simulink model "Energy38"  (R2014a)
settings: Solver=VariableStepDiscrete  StartTime=0.0  StopTime=0.1  RelTol=1e-3
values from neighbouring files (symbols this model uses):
  Gsimulated = Ivertical4'    [main.m]
libraries: fl_lib x56, nesl_utility x29, elec_lib x25

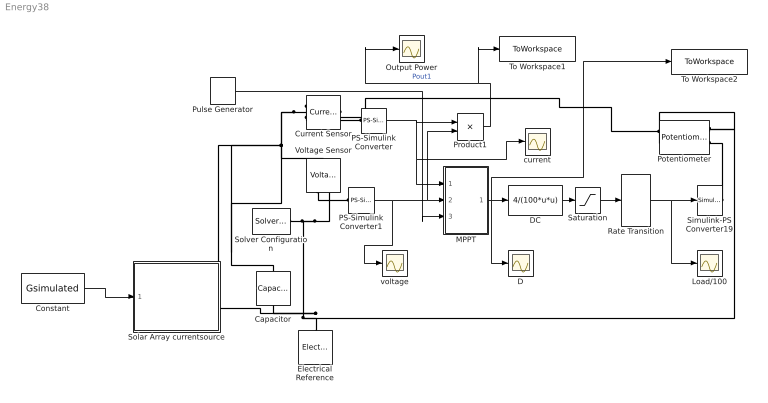
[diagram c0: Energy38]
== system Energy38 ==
  Capacitor : fl_lib/Electrical/Electrical Elements/Capacitor  c=1e-6 F  r=1e-6 Ohm  g=0 1/Ohm  i_specify=off  i_priority=High  i=0 A  v_specify=off  v_priority=High  v=0 V  vc_specify=off  vc_priority=High  vc=0 V
  Constant : Constant  Value=Gsimulated
  Current Sensor : fl_lib/Electrical/Electrical Sensors/Current Sensor
  D : Scope
  DC : Fcn  Expr=4/(100*u*u)
  Electrical Reference : fl_lib/Electrical/Electrical Elements/Electrical Reference
  Load/100 : Scope
  MPPT : Subsystem
  Output Power : Scope
  PS-Simulink Converter : nesl_utility/PS-Simulink Converter  PhysicalDomain=network_engine_domain  SubClassName=ps_output  LeftPortType=input  RightPortType=output  PseudoPeriodic=off  Frequencies=[]  Unit=1  AffineConversion=off
  PS-Simulink Converter1 : nesl_utility/PS-Simulink Converter  PhysicalDomain=network_engine_domain  SubClassName=ps_output  LeftPortType=input  RightPortType=output  PseudoPeriodic=off  Frequencies=[]  Unit=1  AffineConversion=off
  Potentiometer : elec_lib/Passive Devices/Potentiometer  R0=100 Ohm  Rw=0.01 Ohm  Rcenter=200 Ohm  xmin=0  xmax=1  Taper=1  Gradient=1  xminL=0  xmaxL=1  lambda=1  A=1 Ohm
  Product1 : Product
  Pulse Generator : DiscretePulseGenerator  PulseType=Time based  Period=0.3  PulseWidth=0.1
  Rate Transition : RateTransition
  Saturation : Saturate  UpperLimit=1  LowerLimit=0
  Simulink-PS Converter19 : nesl_utility/Simulink-PS Converter  PhysicalDomain=network_engine_domain  SubClassName=ps_input  LeftPortType=input  RightPortType=output  PseudoPeriodic=off  Frequencies=[]  NoiseDistribution=none  NoiseParameters=[]  Unit=1  AffineConversion=off  InputFiltering=off  SimscapeFilterOrder=1  InputFilterTimeConstant=0.001  UdotUserProvided=1
  Solar Array currentsource : Subsystem
  Solver Configuration : nesl_utility/Solver Configuration  PhysicalDomain=network_engine_domain  SubClassName=solver  LeftPortType=input  RightPortType=generic  Accelerate=off  Tones=[]  Harmonics=[]  SimulateNoise=off  Profile=off  UseLocalSampling=off  EnableSwitchedLinearOptims=on  FrequencyDomain=off  UseCCode=off  RelTol=0.001  AbsTol=1e-06  MinStep=1e-09  ToWorkspace=off  DoDC=off  ResidualTolerance=1e-09  UseLocalSolver=on  LocalSolverChoice=NE_BACKWARD_EULER_ADVANCER  LocalSolverSampleTime=1e-4  DoFixedCost=on  MaxNonlinIter=3  MaxModeIter=2  LinearAlgebra=Sparse  DelaysMemoryBudget=1024  AutomaticFiltering=on  FilteringTimeConstant=0.001
  To Workspace1 : ToWorkspace  VariableName=Psimulated  SampleTime=-1
  To Workspace2 : ToWorkspace  VariableName=Dsimulated  SampleTime=-1
  Voltage Sensor : fl_lib/Electrical/Electrical Sensors/Voltage Sensor
  current : Scope
  voltage : Scope
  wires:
  Product1/1 -> Output Power/1, To Workspace1/1  "Pout1"
  DC/1 -> Saturation/1
  Saturation/1 -> Rate Transition/1
  MPPT/1(D) -> To Workspace2/1, D/1, DC/1
  Rate Transition/1 -> Load/100/1, Simulink-PS Converter19/1
  PS-Simulink Converter1/1 -> voltage/1, Product1/2, MPPT/2(V)
  Pulse Generator/1 -> MPPT/3(Control)
  PS-Simulink Converter/1 -> current/1, MPPT/1(I), Product1/1
  Constant/1 -> Solar Array currentsource/1(Gsimulated)
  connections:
  Current Sensor/LConn1 -- Voltage Sensor/LConn1 -- Capacitor/LConn1 -- Solar Array currentsource/RConn1
  Solver Configuration/RConn1 -- Voltage Sensor/RConn2 -- Capacitor/RConn1 -- Solar Array currentsource/RConn2 -- Potentiometer/LConn2 -- Potentiometer/RConn1 -- Electrical Reference/LConn1
  Voltage Sensor/RConn1 -- PS-Simulink Converter1/LConn1
  Current Sensor/RConn1 -- PS-Simulink Converter/LConn1
  Simulink-PS Converter19/RConn1 -- Potentiometer/RConn2
  Potentiometer/LConn1 -- Current Sensor/RConn2

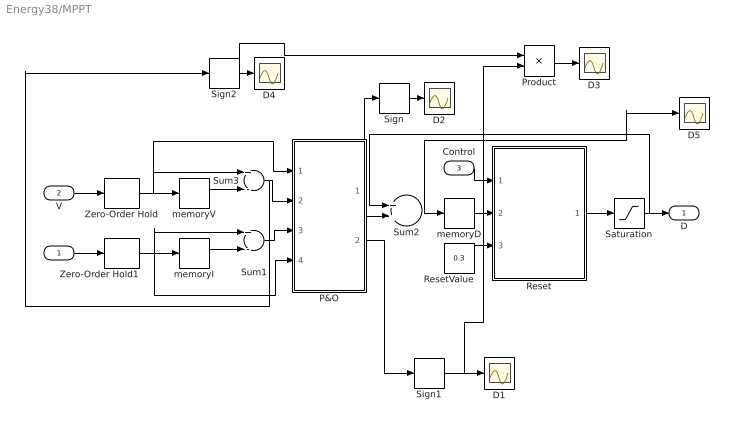
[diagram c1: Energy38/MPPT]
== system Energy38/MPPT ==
  I : Inport
  V : Inport  Port=2
  Control : Inport  Port=3
  D{1..5} (5 alike) : Scope
  P&O : MATLAB Function  TreatAsAtomicUnit=on
  Product : Product
  Reset : MATLAB Function  TreatAsAtomicUnit=on
  ResetValue : Constant  Value=0.3
  Saturation : Saturate  UpperLimit=1  LowerLimit=0
  Sign : Signum
  Sign1 : Signum
  Sign2 : Signum
  Sum1 : Sum  Inputs=+-
  Sum2 : Sum  Inputs=2
  Sum3 : Sum  Inputs=+-
  Zero-Order Hold : ZeroOrderHold  SampleTime=1e-3
  Zero-Order Hold1 : ZeroOrderHold  SampleTime=1e-3
  memoryD : Memory  X0=0.3  InheritSampleTime=on
  memoryI : Memory  InheritSampleTime=on
  memoryV : Memory  InheritSampleTime=on
  D : Outport
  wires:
  Sum2/1 -> D5/1, memoryD/1
  V/1 -> Zero-Order Hold/1
  I/1 -> Zero-Order Hold1/1
  Zero-Order Hold/1 -> P&O/1(V), Sum3/1, memoryV/1
  memoryV/1 -> Sum3/2
  Zero-Order Hold1/1 -> Sum1/1, P&O/4(I), memoryI/1
  memoryI/1 -> Sum1/2
  Saturation/1 -> Sum2/1, D/1
  Sum3/1 -> Sign2/1, P&O/2(dV)
  Sum1/1 -> P&O/3(dI)
  P&O/1(dD) -> Sum2/2, Sign/1
  ResetValue/1 -> Reset/3(ResetValue)
  memoryD/1 -> Reset/2(in)
  Reset/1(out) -> Saturation/1
  Control/1 -> Reset/1(control)
  Sign/1 -> D2/1
  Sign1/1 -> Product/2, D1/1
  P&O/2(dP) -> Sign1/1
  Product/1 -> D3/1
  Sign2/1 -> Product/1, D4/1

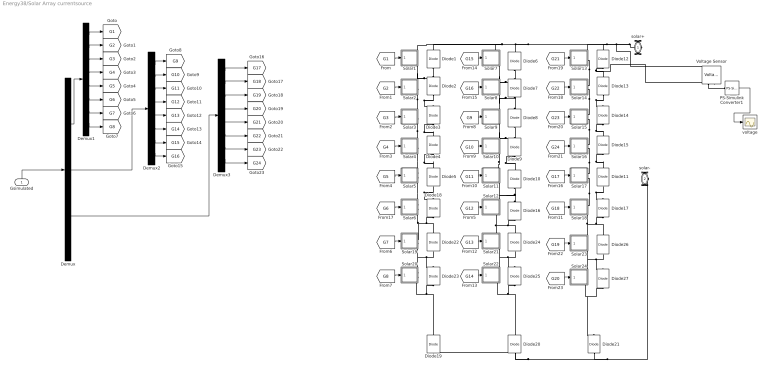
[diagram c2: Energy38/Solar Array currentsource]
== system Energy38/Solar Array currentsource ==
  Gsimulated : Inport
  Demux : Demux  Outputs=3
  Demux1 : Demux  Outputs=8
  Demux2 : Demux  Outputs=8
  Demux3 : Demux  Outputs=8
  Diode{1..27} (27 alike) : fl_lib/Electrical/Electrical Elements/Diode  Vf=0.1 mV  Ron=0.6 Ohm  Goff=1e-10 1/Ohm  i_specify=off  i_priority=High  i=0 A  v_specify=off  v_priority=High  v=0 V
  PS-Simulink Converter1 : nesl_utility/PS-Simulink Converter  PhysicalDomain=network_engine_domain  SubClassName=ps_output  LeftPortType=input  RightPortType=output  PseudoPeriodic=off  Frequencies=[]  Unit=1  AffineConversion=off
  Solar1 : Subsystem
  Solar10 : Subsystem
  Solar11 : Subsystem
  Solar12 : Subsystem
  Solar13 : Subsystem
  Solar14 : Subsystem
  Solar15 : Subsystem
  Solar16 : Subsystem
  Solar17 : Subsystem
  Solar18 : Subsystem
  Solar19 : Subsystem
  Solar2 : Subsystem
  Solar20 : Subsystem
  Solar21 : Subsystem
  Solar22 : Subsystem
  Solar23 : Subsystem
  Solar24 : Subsystem
  Solar3 : Subsystem
  Solar4 : Subsystem
  Solar5 : Subsystem
  Solar6 : Subsystem
  Solar7 : Subsystem
  Solar8 : Subsystem
  Solar9 : Subsystem
  Voltage Sensor : fl_lib/Electrical/Electrical Sensors/Voltage Sensor
  voltage : Scope
  solar+ : PMIOPort  Port=1  Side=Right
  solar- : PMIOPort  Port=2  Side=Right
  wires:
  [G1] -> Solar1/1(G)
  [G2] -> Solar2/1(G)
  [G3] -> Solar3/1(G)
  Gsimulated/1 -> Demux/1
  [G4] -> Solar4/1(G)
  [G9] -> Solar9/1(G)
  [G10] -> Solar10/1(G)
  [G11] -> Solar11/1(G)
  [G17] -> Solar17/1(G)
  Demux/1 -> Demux1/1
  Demux1/1 -> [G1]
  Demux1/2 -> [G2]
  Demux1/3 -> [G3]
  Demux1/4 -> [G4]
  Demux1/5 -> [G5]
  Demux1/6 -> [G6]
  Demux/2 -> Demux2/1
  Demux/3 -> Demux3/1
  [G6] -> Solar6/1(G)
  [G12] -> Solar12/1(G)
  [G18] -> Solar18/1(G)
  [G5] -> Solar5/1(G)
  PS-Simulink Converter1/1 -> voltage/1
  Demux1/7 -> [G7]
  Demux1/8 -> [G8]
  Demux2/1 -> [G9]
  Demux2/2 -> [G10]
  Demux2/3 -> [G11]
  Demux2/4 -> [G12]
  Demux2/5 -> [G13]
  Demux2/6 -> [G14]
  Demux2/7 -> [G15]
  Demux2/8 -> [G16]
  Demux3/1 -> [G17]
  Demux3/2 -> [G18]
  Demux3/3 -> [G19]
  Demux3/4 -> [G20]
  Demux3/5 -> [G21]
  Demux3/6 -> [G22]
  Demux3/7 -> [G23]
  Demux3/8 -> [G24]
  [G7] -> Solar19/1(G)
  [G8] -> Solar20/1(G)
  [G19] -> Solar23/1(G)
  [G20] -> Solar24/1(G)
  [G13] -> Solar21/1(G)
  [G14] -> Solar22/1(G)
  [G15] -> Solar7/1(G)
  [G16] -> Solar8/1(G)
  [G21] -> Solar13/1(G)
  [G22] -> Solar14/1(G)
  [G23] -> Solar15/1(G)
  [G24] -> Solar16/1(G)
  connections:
  Solar15/RConn2 -- Diode15/RConn1 -- Diode14/LConn1 -- Solar16/RConn1
  Solar13/RConn2 -- Voltage Sensor/RConn2 -- Diode13/RConn1 -- Diode12/LConn1 -- Solar14/RConn1
  Diode7/LConn1 -- Diode8/RConn1 -- Solar9/RConn1 -- Solar8/RConn2
  Solar4/RConn2 -- Diode5/RConn1 -- Diode4/LConn1 -- Solar5/RConn1
  solar+/RConn1 -- Solar1/RConn1 -- Diode1/RConn1 -- Solar7/RConn1 -- Diode6/RConn1 -- Solar13/RConn1 -- Diode12/RConn1 -- Voltage Sensor/LConn1
  Diode2/RConn1 -- Diode1/LConn1 -- Solar1/RConn2 -- Solar2/RConn1
  Diode7/RConn1 -- Diode6/LConn1 -- Solar7/RConn2 -- Solar8/RConn1
  Solar14/RConn2 -- Diode13/LConn1 -- Diode14/RConn1 -- Solar15/RConn1
  Solar2/RConn2 -- Diode2/LConn1 -- Diode3/RConn1 -- Solar3/RConn1
  Solar3/RConn2 -- Diode4/RConn1 -- Diode3/LConn1 -- Solar4/RConn1
  Diode9/RConn1 -- Diode8/LConn1 -- Solar9/RConn2 -- Solar10/RConn1
  Solar17/RConn1 -- Diode11/RConn1 -- Diode15/LConn1 -- Solar16/RConn2
  Solar10/RConn2 -- Solar11/RConn1 -- Diode10/RConn1 -- Diode9/LConn1
  Diode16/RConn1 -- Diode10/LConn1 -- Solar11/RConn2 -- Solar12/RConn1
  Solar6/RConn1 -- Diode5/LConn1 -- Diode18/RConn1 -- Solar5/RConn2
  Solar12/RConn2 -- Solar21/RConn1 -- Diode24/RConn1 -- Diode16/LConn1
  Solar18/RConn1 -- Diode11/LConn1 -- Diode17/RConn1 -- Solar17/RConn2
  solar-/RConn1 -- Diode21/LConn1 -- Diode20/LConn1 -- Diode19/LConn1
  Solar18/RConn2 -- Solar23/RConn1 -- Diode17/LConn1 -- Diode26/RConn1
  Voltage Sensor/RConn1 -- PS-Simulink Converter1/LConn1
  Solar6/RConn2 -- Solar19/RConn1 -- Diode22/RConn1 -- Diode18/LConn1
  Solar20/RConn2 -- Diode19/RConn1 -- Diode23/LConn1
  Solar19/RConn2 -- Diode22/LConn1 -- Diode23/RConn1 -- Solar20/RConn1
  Solar22/RConn2 -- Diode20/RConn1 -- Diode25/LConn1
  Solar21/RConn2 -- Diode24/LConn1 -- Diode25/RConn1 -- Solar22/RConn1
  Solar24/RConn2 -- Diode27/LConn1 -- Diode21/RConn1
  Solar23/RConn2 -- Diode26/LConn1 -- Diode27/RConn1 -- Solar24/RConn1

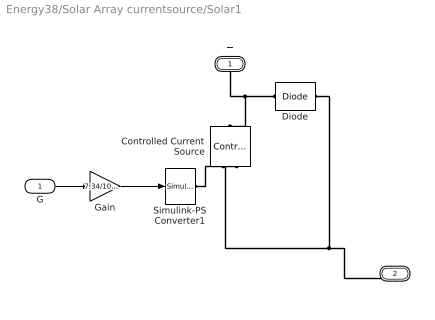
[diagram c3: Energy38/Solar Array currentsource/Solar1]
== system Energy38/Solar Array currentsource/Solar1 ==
  G : Inport
  Controlled Current Source : fl_lib/Electrical/Electrical Sources/Controlled Current Source
  Diode : elec_lib/Semiconductor Devices/Diode  ModelType=3  Vf=0.6 V  Ron=0.3 Ohm  Goff=1e-8 S  Rz=0.3 Ohm  Vz=50 V  C_PWL=5 pF  prmExp=2  I12=[ 0.0137 0.545 ] A  V12=[ 0.6 0.7 ] V  I1=0.0137 A  V1=0.6 V  RS=0.01 Ohm  IS=1.2614e-07 A  Tmeas=25 C  ec=117.5087  BV=Inf V  C_param=1  CJ0=5 pF  VJ=1 V  Mgrad=0.5  Vvec=[ 0.1 10 100 ] V  Cvec=[ 3.5 1 0.4 ] pF  FC=0.5  Q_param=1  Irrm=-7.15 A  iF=4 A  didt=-750 A/us  trr=115 ns  TT=50 ns  tau=100 ns  T_param=1  IS_T2=1.25e-7 A  I1_T2=0.245 A  V1_T2=0.5 V  Tmeas2=125 C  EG_param=1  EG=1.11 eV  XTI_param=1  XTI=3  dBVdT=0 V/K  Tdevice=25 C  Rth=[ 0 10 ] K/W  thermal_mass_parameterization=1  thermal_mass=[ 0 1 ] J/K  thermal_time_constant=[ 0 10 ] s  thermal_mass_initial_temperatures=[ 25 25 ] C
  Gain : Gain  Gain=7.34/1000
  Simulink-PS Converter1 : nesl_utility/Simulink-PS Converter  PhysicalDomain=network_engine_domain  SubClassName=ps_input  LeftPortType=input  RightPortType=output  PseudoPeriodic=off  Frequencies=[]  NoiseDistribution=none  NoiseParameters=[]  Unit=1  AffineConversion=off  InputFiltering=off  SimscapeFilterOrder=1  InputFilterTimeConstant=0.001  UdotUserProvided=1
  + : PMIOPort  Port=1  Side=Right
  - : PMIOPort  Port=2  Side=Right
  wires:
  G/1 -> Gain/1
  Gain/1 -> Simulink-PS Converter1/1
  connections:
  Simulink-PS Converter1/RConn1 -- Controlled Current Source/RConn1
  Diode/RConn1 -- -/RConn1 -- Controlled Current Source/RConn2
  Diode/LConn1 -- Controlled Current Source/LConn1 -- +/RConn1

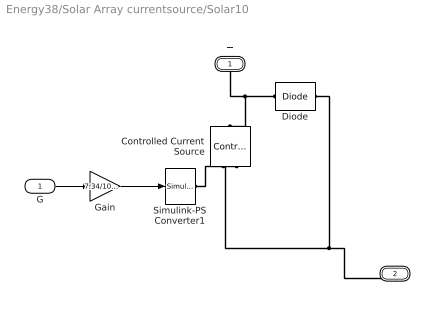
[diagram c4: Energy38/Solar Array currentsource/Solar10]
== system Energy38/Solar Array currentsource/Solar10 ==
  G : Inport
  Controlled Current Source : fl_lib/Electrical/Electrical Sources/Controlled Current Source
  Diode : elec_lib/Semiconductor Devices/Diode  ModelType=3  Vf=0.6 V  Ron=0.3 Ohm  Goff=1e-8 S  Rz=0.3 Ohm  Vz=50 V  C_PWL=5 pF  prmExp=2  I12=[ 0.0137 0.545 ] A  V12=[ 0.6 0.7 ] V  I1=0.0137 A  V1=0.6 V  RS=0.01 Ohm  IS=1.2614e-07 A  Tmeas=25 C  ec=117.5087  BV=Inf V  C_param=1  CJ0=5 pF  VJ=1 V  Mgrad=0.5  Vvec=[ 0.1 10 100 ] V  Cvec=[ 3.5 1 0.4 ] pF  FC=0.5  Q_param=1  Irrm=-7.15 A  iF=4 A  didt=-750 A/us  trr=115 ns  TT=50 ns  tau=100 ns  T_param=1  IS_T2=1.25e-7 A  I1_T2=0.245 A  V1_T2=0.5 V  Tmeas2=125 C  EG_param=1  EG=1.11 eV  XTI_param=1  XTI=3  dBVdT=0 V/K  Tdevice=25 C  Rth=[ 0 10 ] K/W  thermal_mass_parameterization=1  thermal_mass=[ 0 1 ] J/K  thermal_time_constant=[ 0 10 ] s  thermal_mass_initial_temperatures=[ 25 25 ] C
  Gain : Gain  Gain=7.34/1000
  Simulink-PS Converter1 : nesl_utility/Simulink-PS Converter  PhysicalDomain=network_engine_domain  SubClassName=ps_input  LeftPortType=input  RightPortType=output  PseudoPeriodic=off  Frequencies=[]  NoiseDistribution=none  NoiseParameters=[]  Unit=1  AffineConversion=off  InputFiltering=off  SimscapeFilterOrder=1  InputFilterTimeConstant=0.001  UdotUserProvided=1
  + : PMIOPort  Port=1  Side=Right
  - : PMIOPort  Port=2  Side=Right
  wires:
  G/1 -> Gain/1
  Gain/1 -> Simulink-PS Converter1/1
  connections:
  Simulink-PS Converter1/RConn1 -- Controlled Current Source/RConn1
  Diode/RConn1 -- -/RConn1 -- Controlled Current Source/RConn2
  Diode/LConn1 -- Controlled Current Source/LConn1 -- +/RConn1

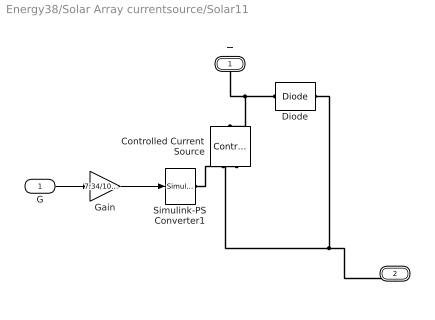
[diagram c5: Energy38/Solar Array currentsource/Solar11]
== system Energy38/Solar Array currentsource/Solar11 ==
  G : Inport
  Controlled Current Source : fl_lib/Electrical/Electrical Sources/Controlled Current Source
  Diode : elec_lib/Semiconductor Devices/Diode  ModelType=3  Vf=0.6 V  Ron=0.3 Ohm  Goff=1e-8 S  Rz=0.3 Ohm  Vz=50 V  C_PWL=5 pF  prmExp=2  I12=[ 0.0137 0.545 ] A  V12=[ 0.6 0.7 ] V  I1=0.0137 A  V1=0.6 V  RS=0.01 Ohm  IS=1.2614e-07 A  Tmeas=25 C  ec=117.5087  BV=Inf V  C_param=1  CJ0=5 pF  VJ=1 V  Mgrad=0.5  Vvec=[ 0.1 10 100 ] V  Cvec=[ 3.5 1 0.4 ] pF  FC=0.5  Q_param=1  Irrm=-7.15 A  iF=4 A  didt=-750 A/us  trr=115 ns  TT=50 ns  tau=100 ns  T_param=1  IS_T2=1.25e-7 A  I1_T2=0.245 A  V1_T2=0.5 V  Tmeas2=125 C  EG_param=1  EG=1.11 eV  XTI_param=1  XTI=3  dBVdT=0 V/K  Tdevice=25 C  Rth=[ 0 10 ] K/W  thermal_mass_parameterization=1  thermal_mass=[ 0 1 ] J/K  thermal_time_constant=[ 0 10 ] s  thermal_mass_initial_temperatures=[ 25 25 ] C
  Gain : Gain  Gain=7.34/1000
  Simulink-PS Converter1 : nesl_utility/Simulink-PS Converter  PhysicalDomain=network_engine_domain  SubClassName=ps_input  LeftPortType=input  RightPortType=output  PseudoPeriodic=off  Frequencies=[]  NoiseDistribution=none  NoiseParameters=[]  Unit=1  AffineConversion=off  InputFiltering=off  SimscapeFilterOrder=1  InputFilterTimeConstant=0.001  UdotUserProvided=1
  + : PMIOPort  Port=1  Side=Right
  - : PMIOPort  Port=2  Side=Right
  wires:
  G/1 -> Gain/1
  Gain/1 -> Simulink-PS Converter1/1
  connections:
  Simulink-PS Converter1/RConn1 -- Controlled Current Source/RConn1
  Diode/RConn1 -- -/RConn1 -- Controlled Current Source/RConn2
  Diode/LConn1 -- Controlled Current Source/LConn1 -- +/RConn1

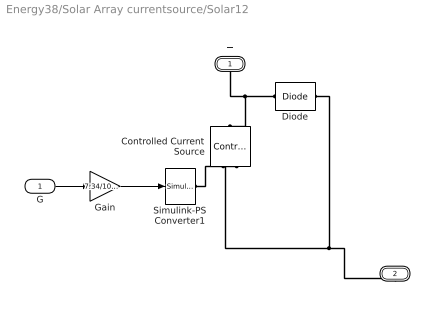
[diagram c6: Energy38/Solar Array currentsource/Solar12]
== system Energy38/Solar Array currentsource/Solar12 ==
  G : Inport
  Controlled Current Source : fl_lib/Electrical/Electrical Sources/Controlled Current Source
  Diode : elec_lib/Semiconductor Devices/Diode  ModelType=3  Vf=0.6 V  Ron=0.3 Ohm  Goff=1e-8 S  Rz=0.3 Ohm  Vz=50 V  C_PWL=5 pF  prmExp=2  I12=[ 0.0137 0.545 ] A  V12=[ 0.6 0.7 ] V  I1=0.0137 A  V1=0.6 V  RS=0.01 Ohm  IS=1.2614e-07 A  Tmeas=25 C  ec=117.5087  BV=Inf V  C_param=1  CJ0=5 pF  VJ=1 V  Mgrad=0.5  Vvec=[ 0.1 10 100 ] V  Cvec=[ 3.5 1 0.4 ] pF  FC=0.5  Q_param=1  Irrm=-7.15 A  iF=4 A  didt=-750 A/us  trr=115 ns  TT=50 ns  tau=100 ns  T_param=1  IS_T2=1.25e-7 A  I1_T2=0.245 A  V1_T2=0.5 V  Tmeas2=125 C  EG_param=1  EG=1.11 eV  XTI_param=1  XTI=3  dBVdT=0 V/K  Tdevice=25 C  Rth=[ 0 10 ] K/W  thermal_mass_parameterization=1  thermal_mass=[ 0 1 ] J/K  thermal_time_constant=[ 0 10 ] s  thermal_mass_initial_temperatures=[ 25 25 ] C
  Gain : Gain  Gain=7.34/1000
  Simulink-PS Converter1 : nesl_utility/Simulink-PS Converter  PhysicalDomain=network_engine_domain  SubClassName=ps_input  LeftPortType=input  RightPortType=output  PseudoPeriodic=off  Frequencies=[]  NoiseDistribution=none  NoiseParameters=[]  Unit=1  AffineConversion=off  InputFiltering=off  SimscapeFilterOrder=1  InputFilterTimeConstant=0.001  UdotUserProvided=1
  + : PMIOPort  Port=1  Side=Right
  - : PMIOPort  Port=2  Side=Right
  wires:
  G/1 -> Gain/1
  Gain/1 -> Simulink-PS Converter1/1
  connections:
  Simulink-PS Converter1/RConn1 -- Controlled Current Source/RConn1
  Diode/RConn1 -- -/RConn1 -- Controlled Current Source/RConn2
  Diode/LConn1 -- Controlled Current Source/LConn1 -- +/RConn1

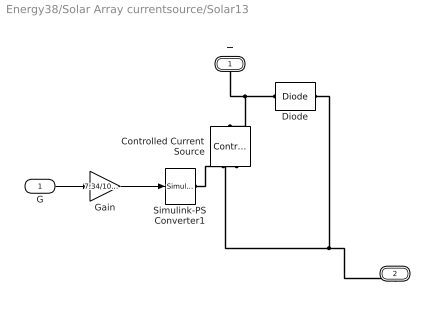
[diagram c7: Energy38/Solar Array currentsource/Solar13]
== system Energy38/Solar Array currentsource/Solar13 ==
  G : Inport
  Controlled Current Source : fl_lib/Electrical/Electrical Sources/Controlled Current Source
  Diode : elec_lib/Semiconductor Devices/Diode  ModelType=3  Vf=0.6 V  Ron=0.3 Ohm  Goff=1e-8 S  Rz=0.3 Ohm  Vz=50 V  C_PWL=5 pF  prmExp=2  I12=[ 0.0137 0.545 ] A  V12=[ 0.6 0.7 ] V  I1=0.0137 A  V1=0.6 V  RS=0.01 Ohm  IS=1.2614e-07 A  Tmeas=25 C  ec=117.5087  BV=Inf V  C_param=1  CJ0=5 pF  VJ=1 V  Mgrad=0.5  Vvec=[ 0.1 10 100 ] V  Cvec=[ 3.5 1 0.4 ] pF  FC=0.5  Q_param=1  Irrm=-7.15 A  iF=4 A  didt=-750 A/us  trr=115 ns  TT=50 ns  tau=100 ns  T_param=1  IS_T2=1.25e-7 A  I1_T2=0.245 A  V1_T2=0.5 V  Tmeas2=125 C  EG_param=1  EG=1.11 eV  XTI_param=1  XTI=3  dBVdT=0 V/K  Tdevice=25 C  Rth=[ 0 10 ] K/W  thermal_mass_parameterization=1  thermal_mass=[ 0 1 ] J/K  thermal_time_constant=[ 0 10 ] s  thermal_mass_initial_temperatures=[ 25 25 ] C
  Gain : Gain  Gain=7.34/1000
  Simulink-PS Converter1 : nesl_utility/Simulink-PS Converter  PhysicalDomain=network_engine_domain  SubClassName=ps_input  LeftPortType=input  RightPortType=output  PseudoPeriodic=off  Frequencies=[]  NoiseDistribution=none  NoiseParameters=[]  Unit=1  AffineConversion=off  InputFiltering=off  SimscapeFilterOrder=1  InputFilterTimeConstant=0.001  UdotUserProvided=1
  + : PMIOPort  Port=1  Side=Right
  - : PMIOPort  Port=2  Side=Right
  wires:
  G/1 -> Gain/1
  Gain/1 -> Simulink-PS Converter1/1
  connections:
  Simulink-PS Converter1/RConn1 -- Controlled Current Source/RConn1
  Diode/RConn1 -- -/RConn1 -- Controlled Current Source/RConn2
  Diode/LConn1 -- Controlled Current Source/LConn1 -- +/RConn1

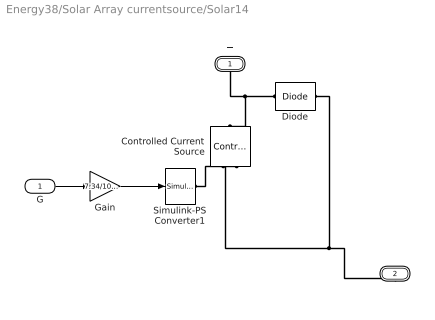
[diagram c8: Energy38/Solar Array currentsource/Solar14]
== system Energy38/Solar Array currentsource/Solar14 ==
  G : Inport
  Controlled Current Source : fl_lib/Electrical/Electrical Sources/Controlled Current Source
  Diode : elec_lib/Semiconductor Devices/Diode  ModelType=3  Vf=0.6 V  Ron=0.3 Ohm  Goff=1e-8 S  Rz=0.3 Ohm  Vz=50 V  C_PWL=5 pF  prmExp=2  I12=[ 0.0137 0.545 ] A  V12=[ 0.6 0.7 ] V  I1=0.0137 A  V1=0.6 V  RS=0.01 Ohm  IS=1.2614e-07 A  Tmeas=25 C  ec=117.5087  BV=Inf V  C_param=1  CJ0=5 pF  VJ=1 V  Mgrad=0.5  Vvec=[ 0.1 10 100 ] V  Cvec=[ 3.5 1 0.4 ] pF  FC=0.5  Q_param=1  Irrm=-7.15 A  iF=4 A  didt=-750 A/us  trr=115 ns  TT=50 ns  tau=100 ns  T_param=1  IS_T2=1.25e-7 A  I1_T2=0.245 A  V1_T2=0.5 V  Tmeas2=125 C  EG_param=1  EG=1.11 eV  XTI_param=1  XTI=3  dBVdT=0 V/K  Tdevice=25 C  Rth=[ 0 10 ] K/W  thermal_mass_parameterization=1  thermal_mass=[ 0 1 ] J/K  thermal_time_constant=[ 0 10 ] s  thermal_mass_initial_temperatures=[ 25 25 ] C
  Gain : Gain  Gain=7.34/1000
  Simulink-PS Converter1 : nesl_utility/Simulink-PS Converter  PhysicalDomain=network_engine_domain  SubClassName=ps_input  LeftPortType=input  RightPortType=output  PseudoPeriodic=off  Frequencies=[]  NoiseDistribution=none  NoiseParameters=[]  Unit=1  AffineConversion=off  InputFiltering=off  SimscapeFilterOrder=1  InputFilterTimeConstant=0.001  UdotUserProvided=1
  + : PMIOPort  Port=1  Side=Right
  - : PMIOPort  Port=2  Side=Right
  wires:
  G/1 -> Gain/1
  Gain/1 -> Simulink-PS Converter1/1
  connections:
  Simulink-PS Converter1/RConn1 -- Controlled Current Source/RConn1
  Diode/RConn1 -- -/RConn1 -- Controlled Current Source/RConn2
  Diode/LConn1 -- Controlled Current Source/LConn1 -- +/RConn1

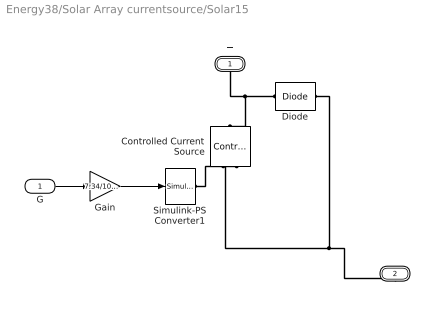
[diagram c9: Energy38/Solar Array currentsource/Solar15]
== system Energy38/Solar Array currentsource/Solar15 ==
  G : Inport
  Controlled Current Source : fl_lib/Electrical/Electrical Sources/Controlled Current Source
  Diode : elec_lib/Semiconductor Devices/Diode  ModelType=3  Vf=0.6 V  Ron=0.3 Ohm  Goff=1e-8 S  Rz=0.3 Ohm  Vz=50 V  C_PWL=5 pF  prmExp=2  I12=[ 0.0137 0.545 ] A  V12=[ 0.6 0.7 ] V  I1=0.0137 A  V1=0.6 V  RS=0.01 Ohm  IS=1.2614e-07 A  Tmeas=25 C  ec=117.5087  BV=Inf V  C_param=1  CJ0=5 pF  VJ=1 V  Mgrad=0.5  Vvec=[ 0.1 10 100 ] V  Cvec=[ 3.5 1 0.4 ] pF  FC=0.5  Q_param=1  Irrm=-7.15 A  iF=4 A  didt=-750 A/us  trr=115 ns  TT=50 ns  tau=100 ns  T_param=1  IS_T2=1.25e-7 A  I1_T2=0.245 A  V1_T2=0.5 V  Tmeas2=125 C  EG_param=1  EG=1.11 eV  XTI_param=1  XTI=3  dBVdT=0 V/K  Tdevice=25 C  Rth=[ 0 10 ] K/W  thermal_mass_parameterization=1  thermal_mass=[ 0 1 ] J/K  thermal_time_constant=[ 0 10 ] s  thermal_mass_initial_temperatures=[ 25 25 ] C
  Gain : Gain  Gain=7.34/1000
  Simulink-PS Converter1 : nesl_utility/Simulink-PS Converter  PhysicalDomain=network_engine_domain  SubClassName=ps_input  LeftPortType=input  RightPortType=output  PseudoPeriodic=off  Frequencies=[]  NoiseDistribution=none  NoiseParameters=[]  Unit=1  AffineConversion=off  InputFiltering=off  SimscapeFilterOrder=1  InputFilterTimeConstant=0.001  UdotUserProvided=1
  + : PMIOPort  Port=1  Side=Right
  - : PMIOPort  Port=2  Side=Right
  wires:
  G/1 -> Gain/1
  Gain/1 -> Simulink-PS Converter1/1
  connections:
  Simulink-PS Converter1/RConn1 -- Controlled Current Source/RConn1
  Diode/RConn1 -- -/RConn1 -- Controlled Current Source/RConn2
  Diode/LConn1 -- Controlled Current Source/LConn1 -- +/RConn1

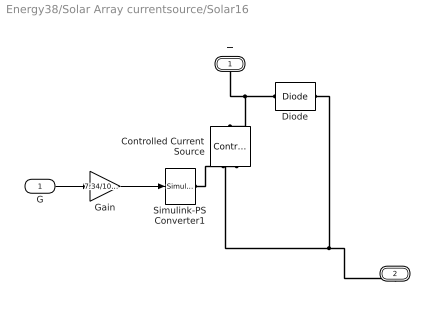
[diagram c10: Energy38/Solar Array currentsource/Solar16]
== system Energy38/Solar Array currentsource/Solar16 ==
  G : Inport
  Controlled Current Source : fl_lib/Electrical/Electrical Sources/Controlled Current Source
  Diode : elec_lib/Semiconductor Devices/Diode  ModelType=3  Vf=0.6 V  Ron=0.3 Ohm  Goff=1e-8 S  Rz=0.3 Ohm  Vz=50 V  C_PWL=5 pF  prmExp=2  I12=[ 0.0137 0.545 ] A  V12=[ 0.6 0.7 ] V  I1=0.0137 A  V1=0.6 V  RS=0.01 Ohm  IS=1.2614e-07 A  Tmeas=25 C  ec=117.5087  BV=Inf V  C_param=1  CJ0=5 pF  VJ=1 V  Mgrad=0.5  Vvec=[ 0.1 10 100 ] V  Cvec=[ 3.5 1 0.4 ] pF  FC=0.5  Q_param=1  Irrm=-7.15 A  iF=4 A  didt=-750 A/us  trr=115 ns  TT=50 ns  tau=100 ns  T_param=1  IS_T2=1.25e-7 A  I1_T2=0.245 A  V1_T2=0.5 V  Tmeas2=125 C  EG_param=1  EG=1.11 eV  XTI_param=1  XTI=3  dBVdT=0 V/K  Tdevice=25 C  Rth=[ 0 10 ] K/W  thermal_mass_parameterization=1  thermal_mass=[ 0 1 ] J/K  thermal_time_constant=[ 0 10 ] s  thermal_mass_initial_temperatures=[ 25 25 ] C
  Gain : Gain  Gain=7.34/1000
  Simulink-PS Converter1 : nesl_utility/Simulink-PS Converter  PhysicalDomain=network_engine_domain  SubClassName=ps_input  LeftPortType=input  RightPortType=output  PseudoPeriodic=off  Frequencies=[]  NoiseDistribution=none  NoiseParameters=[]  Unit=1  AffineConversion=off  InputFiltering=off  SimscapeFilterOrder=1  InputFilterTimeConstant=0.001  UdotUserProvided=1
  + : PMIOPort  Port=1  Side=Right
  - : PMIOPort  Port=2  Side=Right
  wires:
  G/1 -> Gain/1
  Gain/1 -> Simulink-PS Converter1/1
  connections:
  Simulink-PS Converter1/RConn1 -- Controlled Current Source/RConn1
  Diode/RConn1 -- -/RConn1 -- Controlled Current Source/RConn2
  Diode/LConn1 -- Controlled Current Source/LConn1 -- +/RConn1

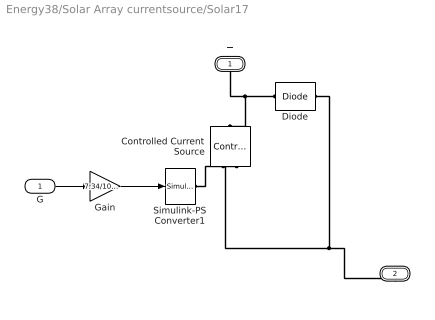
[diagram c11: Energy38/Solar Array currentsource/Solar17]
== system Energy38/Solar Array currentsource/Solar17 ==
  G : Inport
  Controlled Current Source : fl_lib/Electrical/Electrical Sources/Controlled Current Source
  Diode : elec_lib/Semiconductor Devices/Diode  ModelType=3  Vf=0.6 V  Ron=0.3 Ohm  Goff=1e-8 S  Rz=0.3 Ohm  Vz=50 V  C_PWL=5 pF  prmExp=2  I12=[ 0.0137 0.545 ] A  V12=[ 0.6 0.7 ] V  I1=0.0137 A  V1=0.6 V  RS=0.01 Ohm  IS=1.2614e-07 A  Tmeas=25 C  ec=117.5087  BV=Inf V  C_param=1  CJ0=5 pF  VJ=1 V  Mgrad=0.5  Vvec=[ 0.1 10 100 ] V  Cvec=[ 3.5 1 0.4 ] pF  FC=0.5  Q_param=1  Irrm=-7.15 A  iF=4 A  didt=-750 A/us  trr=115 ns  TT=50 ns  tau=100 ns  T_param=1  IS_T2=1.25e-7 A  I1_T2=0.245 A  V1_T2=0.5 V  Tmeas2=125 C  EG_param=1  EG=1.11 eV  XTI_param=1  XTI=3  dBVdT=0 V/K  Tdevice=25 C  Rth=[ 0 10 ] K/W  thermal_mass_parameterization=1  thermal_mass=[ 0 1 ] J/K  thermal_time_constant=[ 0 10 ] s  thermal_mass_initial_temperatures=[ 25 25 ] C
  Gain : Gain  Gain=7.34/1000
  Simulink-PS Converter1 : nesl_utility/Simulink-PS Converter  PhysicalDomain=network_engine_domain  SubClassName=ps_input  LeftPortType=input  RightPortType=output  PseudoPeriodic=off  Frequencies=[]  NoiseDistribution=none  NoiseParameters=[]  Unit=1  AffineConversion=off  InputFiltering=off  SimscapeFilterOrder=1  InputFilterTimeConstant=0.001  UdotUserProvided=1
  + : PMIOPort  Port=1  Side=Right
  - : PMIOPort  Port=2  Side=Right
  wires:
  G/1 -> Gain/1
  Gain/1 -> Simulink-PS Converter1/1
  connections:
  Simulink-PS Converter1/RConn1 -- Controlled Current Source/RConn1
  Diode/RConn1 -- -/RConn1 -- Controlled Current Source/RConn2
  Diode/LConn1 -- Controlled Current Source/LConn1 -- +/RConn1

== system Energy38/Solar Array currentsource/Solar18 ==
  G : Inport
  Controlled Current Source : fl_lib/Electrical/Electrical Sources/Controlled Current Source
  Diode : elec_lib/Semiconductor Devices/Diode  ModelType=3  Vf=0.6 V  Ron=0.3 Ohm  Goff=1e-8 S  Rz=0.3 Ohm  Vz=50 V  C_PWL=5 pF  prmExp=2  I12=[ 0.0137 0.545 ] A  V12=[ 0.6 0.7 ] V  I1=0.0137 A  V1=0.6 V  RS=0.01 Ohm  IS=1.2614e-07 A  Tmeas=25 C  ec=117.5087  BV=Inf V  C_param=1  CJ0=5 pF  VJ=1 V  Mgrad=0.5  Vvec=[ 0.1 10 100 ] V  Cvec=[ 3.5 1 0.4 ] pF  FC=0.5  Q_param=1  Irrm=-7.15 A  iF=4 A  didt=-750 A/us  trr=115 ns  TT=50 ns  tau=100 ns  T_param=1  IS_T2=1.25e-7 A  I1_T2=0.245 A  V1_T2=0.5 V  Tmeas2=125 C  EG_param=1  EG=1.11 eV  XTI_param=1  XTI=3  dBVdT=0 V/K  Tdevice=25 C  Rth=[ 0 10 ] K/W  thermal_mass_parameterization=1  thermal_mass=[ 0 1 ] J/K  thermal_time_constant=[ 0 10 ] s  thermal_mass_initial_temperatures=[ 25 25 ] C
  Gain : Gain  Gain=7.34/1000
  Simulink-PS Converter1 : nesl_utility/Simulink-PS Converter  PhysicalDomain=network_engine_domain  SubClassName=ps_input  LeftPortType=input  RightPortType=output  PseudoPeriodic=off  Frequencies=[]  NoiseDistribution=none  NoiseParameters=[]  Unit=1  AffineConversion=off  InputFiltering=off  SimscapeFilterOrder=1  InputFilterTimeConstant=0.001  UdotUserProvided=1
  + : PMIOPort  Port=1  Side=Right
  - : PMIOPort  Port=2  Side=Right
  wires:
  G/1 -> Gain/1
  Gain/1 -> Simulink-PS Converter1/1
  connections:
  Simulink-PS Converter1/RConn1 -- Controlled Current Source/RConn1
  Diode/RConn1 -- -/RConn1 -- Controlled Current Source/RConn2
  Diode/LConn1 -- Controlled Current Source/LConn1 -- +/RConn1

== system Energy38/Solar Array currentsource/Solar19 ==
  G : Inport
  Controlled Current Source : fl_lib/Electrical/Electrical Sources/Controlled Current Source
  Diode : elec_lib/Semiconductor Devices/Diode  ModelType=3  Vf=0.6 V  Ron=0.3 Ohm  Goff=1e-8 S  Rz=0.3 Ohm  Vz=50 V  C_PWL=5 pF  prmExp=2  I12=[ 0.0137 0.545 ] A  V12=[ 0.6 0.7 ] V  I1=0.0137 A  V1=0.6 V  RS=0.01 Ohm  IS=1.2614e-07 A  Tmeas=25 C  ec=117.5087  BV=Inf V  C_param=1  CJ0=5 pF  VJ=1 V  Mgrad=0.5  Vvec=[ 0.1 10 100 ] V  Cvec=[ 3.5 1 0.4 ] pF  FC=0.5  Q_param=1  Irrm=-7.15 A  iF=4 A  didt=-750 A/us  trr=115 ns  TT=50 ns  tau=100 ns  T_param=1  IS_T2=1.25e-7 A  I1_T2=0.245 A  V1_T2=0.5 V  Tmeas2=125 C  EG_param=1  EG=1.11 eV  XTI_param=1  XTI=3  dBVdT=0 V/K  Tdevice=25 C  Rth=[ 0 10 ] K/W  thermal_mass_parameterization=1  thermal_mass=[ 0 1 ] J/K  thermal_time_constant=[ 0 10 ] s  thermal_mass_initial_temperatures=[ 25 25 ] C
  Gain : Gain  Gain=7.34/1000
  Simulink-PS Converter1 : nesl_utility/Simulink-PS Converter  PhysicalDomain=network_engine_domain  SubClassName=ps_input  LeftPortType=input  RightPortType=output  PseudoPeriodic=off  Frequencies=[]  NoiseDistribution=none  NoiseParameters=[]  Unit=1  AffineConversion=off  InputFiltering=off  SimscapeFilterOrder=1  InputFilterTimeConstant=0.001  UdotUserProvided=1
  + : PMIOPort  Port=1  Side=Right
  - : PMIOPort  Port=2  Side=Right
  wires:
  G/1 -> Gain/1
  Gain/1 -> Simulink-PS Converter1/1
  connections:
  Simulink-PS Converter1/RConn1 -- Controlled Current Source/RConn1
  Diode/RConn1 -- -/RConn1 -- Controlled Current Source/RConn2
  Diode/LConn1 -- Controlled Current Source/LConn1 -- +/RConn1

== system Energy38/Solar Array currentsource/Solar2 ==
  G : Inport
  Controlled Current Source : fl_lib/Electrical/Electrical Sources/Controlled Current Source
  Diode : elec_lib/Semiconductor Devices/Diode  ModelType=3  Vf=0.6 V  Ron=0.3 Ohm  Goff=1e-8 S  Rz=0.3 Ohm  Vz=50 V  C_PWL=5 pF  prmExp=2  I12=[ 0.0137 0.545 ] A  V12=[ 0.6 0.7 ] V  I1=0.0137 A  V1=0.6 V  RS=0.01 Ohm  IS=1.2614e-07 A  Tmeas=25 C  ec=117.5087  BV=Inf V  C_param=1  CJ0=5 pF  VJ=1 V  Mgrad=0.5  Vvec=[ 0.1 10 100 ] V  Cvec=[ 3.5 1 0.4 ] pF  FC=0.5  Q_param=1  Irrm=-7.15 A  iF=4 A  didt=-750 A/us  trr=115 ns  TT=50 ns  tau=100 ns  T_param=1  IS_T2=1.25e-7 A  I1_T2=0.245 A  V1_T2=0.5 V  Tmeas2=125 C  EG_param=1  EG=1.11 eV  XTI_param=1  XTI=3  dBVdT=0 V/K  Tdevice=25 C  Rth=[ 0 10 ] K/W  thermal_mass_parameterization=1  thermal_mass=[ 0 1 ] J/K  thermal_time_constant=[ 0 10 ] s  thermal_mass_initial_temperatures=[ 25 25 ] C
  Gain : Gain  Gain=7.34/1000
  Simulink-PS Converter1 : nesl_utility/Simulink-PS Converter  PhysicalDomain=network_engine_domain  SubClassName=ps_input  LeftPortType=input  RightPortType=output  PseudoPeriodic=off  Frequencies=[]  NoiseDistribution=none  NoiseParameters=[]  Unit=1  AffineConversion=off  InputFiltering=off  SimscapeFilterOrder=1  InputFilterTimeConstant=0.001  UdotUserProvided=1
  + : PMIOPort  Port=1  Side=Right
  - : PMIOPort  Port=2  Side=Right
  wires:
  G/1 -> Gain/1
  Gain/1 -> Simulink-PS Converter1/1
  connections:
  Simulink-PS Converter1/RConn1 -- Controlled Current Source/RConn1
  Diode/RConn1 -- -/RConn1 -- Controlled Current Source/RConn2
  Diode/LConn1 -- Controlled Current Source/LConn1 -- +/RConn1

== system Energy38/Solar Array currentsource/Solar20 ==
  G : Inport
  Controlled Current Source : fl_lib/Electrical/Electrical Sources/Controlled Current Source
  Diode : elec_lib/Semiconductor Devices/Diode  ModelType=3  Vf=0.6 V  Ron=0.3 Ohm  Goff=1e-8 S  Rz=0.3 Ohm  Vz=50 V  C_PWL=5 pF  prmExp=2  I12=[ 0.0137 0.545 ] A  V12=[ 0.6 0.7 ] V  I1=0.0137 A  V1=0.6 V  RS=0.01 Ohm  IS=1.2614e-07 A  Tmeas=25 C  ec=117.5087  BV=Inf V  C_param=1  CJ0=5 pF  VJ=1 V  Mgrad=0.5  Vvec=[ 0.1 10 100 ] V  Cvec=[ 3.5 1 0.4 ] pF  FC=0.5  Q_param=1  Irrm=-7.15 A  iF=4 A  didt=-750 A/us  trr=115 ns  TT=50 ns  tau=100 ns  T_param=1  IS_T2=1.25e-7 A  I1_T2=0.245 A  V1_T2=0.5 V  Tmeas2=125 C  EG_param=1  EG=1.11 eV  XTI_param=1  XTI=3  dBVdT=0 V/K  Tdevice=25 C  Rth=[ 0 10 ] K/W  thermal_mass_parameterization=1  thermal_mass=[ 0 1 ] J/K  thermal_time_constant=[ 0 10 ] s  thermal_mass_initial_temperatures=[ 25 25 ] C
  Gain : Gain  Gain=7.34/1000
  Simulink-PS Converter1 : nesl_utility/Simulink-PS Converter  PhysicalDomain=network_engine_domain  SubClassName=ps_input  LeftPortType=input  RightPortType=output  PseudoPeriodic=off  Frequencies=[]  NoiseDistribution=none  NoiseParameters=[]  Unit=1  AffineConversion=off  InputFiltering=off  SimscapeFilterOrder=1  InputFilterTimeConstant=0.001  UdotUserProvided=1
  + : PMIOPort  Port=1  Side=Right
  - : PMIOPort  Port=2  Side=Right
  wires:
  G/1 -> Gain/1
  Gain/1 -> Simulink-PS Converter1/1
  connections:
  Simulink-PS Converter1/RConn1 -- Controlled Current Source/RConn1
  Diode/RConn1 -- -/RConn1 -- Controlled Current Source/RConn2
  Diode/LConn1 -- Controlled Current Source/LConn1 -- +/RConn1

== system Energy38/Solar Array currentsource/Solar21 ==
  G : Inport
  Controlled Current Source : fl_lib/Electrical/Electrical Sources/Controlled Current Source
  Diode : elec_lib/Semiconductor Devices/Diode  ModelType=3  Vf=0.6 V  Ron=0.3 Ohm  Goff=1e-8 S  Rz=0.3 Ohm  Vz=50 V  C_PWL=5 pF  prmExp=2  I12=[ 0.0137 0.545 ] A  V12=[ 0.6 0.7 ] V  I1=0.0137 A  V1=0.6 V  RS=0.01 Ohm  IS=1.2614e-07 A  Tmeas=25 C  ec=117.5087  BV=Inf V  C_param=1  CJ0=5 pF  VJ=1 V  Mgrad=0.5  Vvec=[ 0.1 10 100 ] V  Cvec=[ 3.5 1 0.4 ] pF  FC=0.5  Q_param=1  Irrm=-7.15 A  iF=4 A  didt=-750 A/us  trr=115 ns  TT=50 ns  tau=100 ns  T_param=1  IS_T2=1.25e-7 A  I1_T2=0.245 A  V1_T2=0.5 V  Tmeas2=125 C  EG_param=1  EG=1.11 eV  XTI_param=1  XTI=3  dBVdT=0 V/K  Tdevice=25 C  Rth=[ 0 10 ] K/W  thermal_mass_parameterization=1  thermal_mass=[ 0 1 ] J/K  thermal_time_constant=[ 0 10 ] s  thermal_mass_initial_temperatures=[ 25 25 ] C
  Gain : Gain  Gain=7.34/1000
  Simulink-PS Converter1 : nesl_utility/Simulink-PS Converter  PhysicalDomain=network_engine_domain  SubClassName=ps_input  LeftPortType=input  RightPortType=output  PseudoPeriodic=off  Frequencies=[]  NoiseDistribution=none  NoiseParameters=[]  Unit=1  AffineConversion=off  InputFiltering=off  SimscapeFilterOrder=1  InputFilterTimeConstant=0.001  UdotUserProvided=1
  + : PMIOPort  Port=1  Side=Right
  - : PMIOPort  Port=2  Side=Right
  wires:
  G/1 -> Gain/1
  Gain/1 -> Simulink-PS Converter1/1
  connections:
  Simulink-PS Converter1/RConn1 -- Controlled Current Source/RConn1
  Diode/RConn1 -- -/RConn1 -- Controlled Current Source/RConn2
  Diode/LConn1 -- Controlled Current Source/LConn1 -- +/RConn1

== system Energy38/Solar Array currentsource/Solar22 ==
  G : Inport
  Controlled Current Source : fl_lib/Electrical/Electrical Sources/Controlled Current Source
  Diode : elec_lib/Semiconductor Devices/Diode  ModelType=3  Vf=0.6 V  Ron=0.3 Ohm  Goff=1e-8 S  Rz=0.3 Ohm  Vz=50 V  C_PWL=5 pF  prmExp=2  I12=[ 0.0137 0.545 ] A  V12=[ 0.6 0.7 ] V  I1=0.0137 A  V1=0.6 V  RS=0.01 Ohm  IS=1.2614e-07 A  Tmeas=25 C  ec=117.5087  BV=Inf V  C_param=1  CJ0=5 pF  VJ=1 V  Mgrad=0.5  Vvec=[ 0.1 10 100 ] V  Cvec=[ 3.5 1 0.4 ] pF  FC=0.5  Q_param=1  Irrm=-7.15 A  iF=4 A  didt=-750 A/us  trr=115 ns  TT=50 ns  tau=100 ns  T_param=1  IS_T2=1.25e-7 A  I1_T2=0.245 A  V1_T2=0.5 V  Tmeas2=125 C  EG_param=1  EG=1.11 eV  XTI_param=1  XTI=3  dBVdT=0 V/K  Tdevice=25 C  Rth=[ 0 10 ] K/W  thermal_mass_parameterization=1  thermal_mass=[ 0 1 ] J/K  thermal_time_constant=[ 0 10 ] s  thermal_mass_initial_temperatures=[ 25 25 ] C
  Gain : Gain  Gain=7.34/1000
  Simulink-PS Converter1 : nesl_utility/Simulink-PS Converter  PhysicalDomain=network_engine_domain  SubClassName=ps_input  LeftPortType=input  RightPortType=output  PseudoPeriodic=off  Frequencies=[]  NoiseDistribution=none  NoiseParameters=[]  Unit=1  AffineConversion=off  InputFiltering=off  SimscapeFilterOrder=1  InputFilterTimeConstant=0.001  UdotUserProvided=1
  + : PMIOPort  Port=1  Side=Right
  - : PMIOPort  Port=2  Side=Right
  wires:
  G/1 -> Gain/1
  Gain/1 -> Simulink-PS Converter1/1
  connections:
  Simulink-PS Converter1/RConn1 -- Controlled Current Source/RConn1
  Diode/RConn1 -- -/RConn1 -- Controlled Current Source/RConn2
  Diode/LConn1 -- Controlled Current Source/LConn1 -- +/RConn1

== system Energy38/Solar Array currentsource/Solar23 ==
  G : Inport
  Controlled Current Source : fl_lib/Electrical/Electrical Sources/Controlled Current Source
  Diode : elec_lib/Semiconductor Devices/Diode  ModelType=3  Vf=0.6 V  Ron=0.3 Ohm  Goff=1e-8 S  Rz=0.3 Ohm  Vz=50 V  C_PWL=5 pF  prmExp=2  I12=[ 0.0137 0.545 ] A  V12=[ 0.6 0.7 ] V  I1=0.0137 A  V1=0.6 V  RS=0.01 Ohm  IS=1.2614e-07 A  Tmeas=25 C  ec=117.5087  BV=Inf V  C_param=1  CJ0=5 pF  VJ=1 V  Mgrad=0.5  Vvec=[ 0.1 10 100 ] V  Cvec=[ 3.5 1 0.4 ] pF  FC=0.5  Q_param=1  Irrm=-7.15 A  iF=4 A  didt=-750 A/us  trr=115 ns  TT=50 ns  tau=100 ns  T_param=1  IS_T2=1.25e-7 A  I1_T2=0.245 A  V1_T2=0.5 V  Tmeas2=125 C  EG_param=1  EG=1.11 eV  XTI_param=1  XTI=3  dBVdT=0 V/K  Tdevice=25 C  Rth=[ 0 10 ] K/W  thermal_mass_parameterization=1  thermal_mass=[ 0 1 ] J/K  thermal_time_constant=[ 0 10 ] s  thermal_mass_initial_temperatures=[ 25 25 ] C
  Gain : Gain  Gain=7.34/1000
  Simulink-PS Converter1 : nesl_utility/Simulink-PS Converter  PhysicalDomain=network_engine_domain  SubClassName=ps_input  LeftPortType=input  RightPortType=output  PseudoPeriodic=off  Frequencies=[]  NoiseDistribution=none  NoiseParameters=[]  Unit=1  AffineConversion=off  InputFiltering=off  SimscapeFilterOrder=1  InputFilterTimeConstant=0.001  UdotUserProvided=1
  + : PMIOPort  Port=1  Side=Right
  - : PMIOPort  Port=2  Side=Right
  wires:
  G/1 -> Gain/1
  Gain/1 -> Simulink-PS Converter1/1
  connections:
  Simulink-PS Converter1/RConn1 -- Controlled Current Source/RConn1
  Diode/RConn1 -- -/RConn1 -- Controlled Current Source/RConn2
  Diode/LConn1 -- Controlled Current Source/LConn1 -- +/RConn1

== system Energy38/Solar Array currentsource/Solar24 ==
  G : Inport
  Controlled Current Source : fl_lib/Electrical/Electrical Sources/Controlled Current Source
  Diode : elec_lib/Semiconductor Devices/Diode  ModelType=3  Vf=0.6 V  Ron=0.3 Ohm  Goff=1e-8 S  Rz=0.3 Ohm  Vz=50 V  C_PWL=5 pF  prmExp=2  I12=[ 0.0137 0.545 ] A  V12=[ 0.6 0.7 ] V  I1=0.0137 A  V1=0.6 V  RS=0.01 Ohm  IS=1.2614e-07 A  Tmeas=25 C  ec=117.5087  BV=Inf V  C_param=1  CJ0=5 pF  VJ=1 V  Mgrad=0.5  Vvec=[ 0.1 10 100 ] V  Cvec=[ 3.5 1 0.4 ] pF  FC=0.5  Q_param=1  Irrm=-7.15 A  iF=4 A  didt=-750 A/us  trr=115 ns  TT=50 ns  tau=100 ns  T_param=1  IS_T2=1.25e-7 A  I1_T2=0.245 A  V1_T2=0.5 V  Tmeas2=125 C  EG_param=1  EG=1.11 eV  XTI_param=1  XTI=3  dBVdT=0 V/K  Tdevice=25 C  Rth=[ 0 10 ] K/W  thermal_mass_parameterization=1  thermal_mass=[ 0 1 ] J/K  thermal_time_constant=[ 0 10 ] s  thermal_mass_initial_temperatures=[ 25 25 ] C
  Gain : Gain  Gain=7.34/1000
  Simulink-PS Converter1 : nesl_utility/Simulink-PS Converter  PhysicalDomain=network_engine_domain  SubClassName=ps_input  LeftPortType=input  RightPortType=output  PseudoPeriodic=off  Frequencies=[]  NoiseDistribution=none  NoiseParameters=[]  Unit=1  AffineConversion=off  InputFiltering=off  SimscapeFilterOrder=1  InputFilterTimeConstant=0.001  UdotUserProvided=1
  + : PMIOPort  Port=1  Side=Right
  - : PMIOPort  Port=2  Side=Right
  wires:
  G/1 -> Gain/1
  Gain/1 -> Simulink-PS Converter1/1
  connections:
  Simulink-PS Converter1/RConn1 -- Controlled Current Source/RConn1
  Diode/RConn1 -- -/RConn1 -- Controlled Current Source/RConn2
  Diode/LConn1 -- Controlled Current Source/LConn1 -- +/RConn1

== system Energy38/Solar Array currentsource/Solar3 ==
  G : Inport
  Controlled Current Source : fl_lib/Electrical/Electrical Sources/Controlled Current Source
  Diode : elec_lib/Semiconductor Devices/Diode  ModelType=3  Vf=0.6 V  Ron=0.3 Ohm  Goff=1e-8 S  Rz=0.3 Ohm  Vz=50 V  C_PWL=5 pF  prmExp=2  I12=[ 0.0137 0.545 ] A  V12=[ 0.6 0.7 ] V  I1=0.0137 A  V1=0.6 V  RS=0.01 Ohm  IS=1.2614e-07 A  Tmeas=25 C  ec=117.5087  BV=Inf V  C_param=1  CJ0=5 pF  VJ=1 V  Mgrad=0.5  Vvec=[ 0.1 10 100 ] V  Cvec=[ 3.5 1 0.4 ] pF  FC=0.5  Q_param=1  Irrm=-7.15 A  iF=4 A  didt=-750 A/us  trr=115 ns  TT=50 ns  tau=100 ns  T_param=1  IS_T2=1.25e-7 A  I1_T2=0.245 A  V1_T2=0.5 V  Tmeas2=125 C  EG_param=1  EG=1.11 eV  XTI_param=1  XTI=3  dBVdT=0 V/K  Tdevice=25 C  Rth=[ 0 10 ] K/W  thermal_mass_parameterization=1  thermal_mass=[ 0 1 ] J/K  thermal_time_constant=[ 0 10 ] s  thermal_mass_initial_temperatures=[ 25 25 ] C
  Gain : Gain  Gain=7.34/1000
  Simulink-PS Converter1 : nesl_utility/Simulink-PS Converter  PhysicalDomain=network_engine_domain  SubClassName=ps_input  LeftPortType=input  RightPortType=output  PseudoPeriodic=off  Frequencies=[]  NoiseDistribution=none  NoiseParameters=[]  Unit=1  AffineConversion=off  InputFiltering=off  SimscapeFilterOrder=1  InputFilterTimeConstant=0.001  UdotUserProvided=1
  + : PMIOPort  Port=1  Side=Right
  - : PMIOPort  Port=2  Side=Right
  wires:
  G/1 -> Gain/1
  Gain/1 -> Simulink-PS Converter1/1
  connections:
  Simulink-PS Converter1/RConn1 -- Controlled Current Source/RConn1
  Diode/RConn1 -- -/RConn1 -- Controlled Current Source/RConn2
  Diode/LConn1 -- Controlled Current Source/LConn1 -- +/RConn1

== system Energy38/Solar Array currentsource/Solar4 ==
  G : Inport
  Controlled Current Source : fl_lib/Electrical/Electrical Sources/Controlled Current Source
  Diode : elec_lib/Semiconductor Devices/Diode  ModelType=3  Vf=0.6 V  Ron=0.3 Ohm  Goff=1e-8 S  Rz=0.3 Ohm  Vz=50 V  C_PWL=5 pF  prmExp=2  I12=[ 0.0137 0.545 ] A  V12=[ 0.6 0.7 ] V  I1=0.0137 A  V1=0.6 V  RS=0.01 Ohm  IS=1.2614e-07 A  Tmeas=25 C  ec=117.5087  BV=Inf V  C_param=1  CJ0=5 pF  VJ=1 V  Mgrad=0.5  Vvec=[ 0.1 10 100 ] V  Cvec=[ 3.5 1 0.4 ] pF  FC=0.5  Q_param=1  Irrm=-7.15 A  iF=4 A  didt=-750 A/us  trr=115 ns  TT=50 ns  tau=100 ns  T_param=1  IS_T2=1.25e-7 A  I1_T2=0.245 A  V1_T2=0.5 V  Tmeas2=125 C  EG_param=1  EG=1.11 eV  XTI_param=1  XTI=3  dBVdT=0 V/K  Tdevice=25 C  Rth=[ 0 10 ] K/W  thermal_mass_parameterization=1  thermal_mass=[ 0 1 ] J/K  thermal_time_constant=[ 0 10 ] s  thermal_mass_initial_temperatures=[ 25 25 ] C
  Gain : Gain  Gain=7.34/1000
  Simulink-PS Converter1 : nesl_utility/Simulink-PS Converter  PhysicalDomain=network_engine_domain  SubClassName=ps_input  LeftPortType=input  RightPortType=output  PseudoPeriodic=off  Frequencies=[]  NoiseDistribution=none  NoiseParameters=[]  Unit=1  AffineConversion=off  InputFiltering=off  SimscapeFilterOrder=1  InputFilterTimeConstant=0.001  UdotUserProvided=1
  + : PMIOPort  Port=1  Side=Right
  - : PMIOPort  Port=2  Side=Right
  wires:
  G/1 -> Gain/1
  Gain/1 -> Simulink-PS Converter1/1
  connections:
  Simulink-PS Converter1/RConn1 -- Controlled Current Source/RConn1
  Diode/RConn1 -- -/RConn1 -- Controlled Current Source/RConn2
  Diode/LConn1 -- Controlled Current Source/LConn1 -- +/RConn1

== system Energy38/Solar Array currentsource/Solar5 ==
  G : Inport
  Controlled Current Source : fl_lib/Electrical/Electrical Sources/Controlled Current Source
  Diode : elec_lib/Semiconductor Devices/Diode  ModelType=3  Vf=0.6 V  Ron=0.3 Ohm  Goff=1e-8 S  Rz=0.3 Ohm  Vz=50 V  C_PWL=5 pF  prmExp=2  I12=[ 0.0137 0.545 ] A  V12=[ 0.6 0.7 ] V  I1=0.0137 A  V1=0.6 V  RS=0.01 Ohm  IS=1.2614e-07 A  Tmeas=25 C  ec=117.5087  BV=Inf V  C_param=1  CJ0=5 pF  VJ=1 V  Mgrad=0.5  Vvec=[ 0.1 10 100 ] V  Cvec=[ 3.5 1 0.4 ] pF  FC=0.5  Q_param=1  Irrm=-7.15 A  iF=4 A  didt=-750 A/us  trr=115 ns  TT=50 ns  tau=100 ns  T_param=1  IS_T2=1.25e-7 A  I1_T2=0.245 A  V1_T2=0.5 V  Tmeas2=125 C  EG_param=1  EG=1.11 eV  XTI_param=1  XTI=3  dBVdT=0 V/K  Tdevice=25 C  Rth=[ 0 10 ] K/W  thermal_mass_parameterization=1  thermal_mass=[ 0 1 ] J/K  thermal_time_constant=[ 0 10 ] s  thermal_mass_initial_temperatures=[ 25 25 ] C
  Gain : Gain  Gain=7.34/1000
  Simulink-PS Converter1 : nesl_utility/Simulink-PS Converter  PhysicalDomain=network_engine_domain  SubClassName=ps_input  LeftPortType=input  RightPortType=output  PseudoPeriodic=off  Frequencies=[]  NoiseDistribution=none  NoiseParameters=[]  Unit=1  AffineConversion=off  InputFiltering=off  SimscapeFilterOrder=1  InputFilterTimeConstant=0.001  UdotUserProvided=1
  + : PMIOPort  Port=1  Side=Right
  - : PMIOPort  Port=2  Side=Right
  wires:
  G/1 -> Gain/1
  Gain/1 -> Simulink-PS Converter1/1
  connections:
  Simulink-PS Converter1/RConn1 -- Controlled Current Source/RConn1
  Diode/RConn1 -- -/RConn1 -- Controlled Current Source/RConn2
  Diode/LConn1 -- Controlled Current Source/LConn1 -- +/RConn1

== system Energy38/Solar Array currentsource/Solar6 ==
  G : Inport
  Controlled Current Source : fl_lib/Electrical/Electrical Sources/Controlled Current Source
  Diode : elec_lib/Semiconductor Devices/Diode  ModelType=3  Vf=0.6 V  Ron=0.3 Ohm  Goff=1e-8 S  Rz=0.3 Ohm  Vz=50 V  C_PWL=5 pF  prmExp=2  I12=[ 0.0137 0.545 ] A  V12=[ 0.6 0.7 ] V  I1=0.0137 A  V1=0.6 V  RS=0.01 Ohm  IS=1.2614e-07 A  Tmeas=25 C  ec=117.5087  BV=Inf V  C_param=1  CJ0=5 pF  VJ=1 V  Mgrad=0.5  Vvec=[ 0.1 10 100 ] V  Cvec=[ 3.5 1 0.4 ] pF  FC=0.5  Q_param=1  Irrm=-7.15 A  iF=4 A  didt=-750 A/us  trr=115 ns  TT=50 ns  tau=100 ns  T_param=1  IS_T2=1.25e-7 A  I1_T2=0.245 A  V1_T2=0.5 V  Tmeas2=125 C  EG_param=1  EG=1.11 eV  XTI_param=1  XTI=3  dBVdT=0 V/K  Tdevice=25 C  Rth=[ 0 10 ] K/W  thermal_mass_parameterization=1  thermal_mass=[ 0 1 ] J/K  thermal_time_constant=[ 0 10 ] s  thermal_mass_initial_temperatures=[ 25 25 ] C
  Gain : Gain  Gain=7.34/1000
  Simulink-PS Converter1 : nesl_utility/Simulink-PS Converter  PhysicalDomain=network_engine_domain  SubClassName=ps_input  LeftPortType=input  RightPortType=output  PseudoPeriodic=off  Frequencies=[]  NoiseDistribution=none  NoiseParameters=[]  Unit=1  AffineConversion=off  InputFiltering=off  SimscapeFilterOrder=1  InputFilterTimeConstant=0.001  UdotUserProvided=1
  + : PMIOPort  Port=1  Side=Right
  - : PMIOPort  Port=2  Side=Right
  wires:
  G/1 -> Gain/1
  Gain/1 -> Simulink-PS Converter1/1
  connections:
  Simulink-PS Converter1/RConn1 -- Controlled Current Source/RConn1
  Diode/RConn1 -- -/RConn1 -- Controlled Current Source/RConn2
  Diode/LConn1 -- Controlled Current Source/LConn1 -- +/RConn1

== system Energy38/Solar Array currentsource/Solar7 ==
  G : Inport
  Controlled Current Source : fl_lib/Electrical/Electrical Sources/Controlled Current Source
  Diode : elec_lib/Semiconductor Devices/Diode  ModelType=3  Vf=0.6 V  Ron=0.3 Ohm  Goff=1e-8 S  Rz=0.3 Ohm  Vz=50 V  C_PWL=5 pF  prmExp=2  I12=[ 0.0137 0.545 ] A  V12=[ 0.6 0.7 ] V  I1=0.0137 A  V1=0.6 V  RS=0.01 Ohm  IS=1.2614e-07 A  Tmeas=25 C  ec=117.5087  BV=Inf V  C_param=1  CJ0=5 pF  VJ=1 V  Mgrad=0.5  Vvec=[ 0.1 10 100 ] V  Cvec=[ 3.5 1 0.4 ] pF  FC=0.5  Q_param=1  Irrm=-7.15 A  iF=4 A  didt=-750 A/us  trr=115 ns  TT=50 ns  tau=100 ns  T_param=1  IS_T2=1.25e-7 A  I1_T2=0.245 A  V1_T2=0.5 V  Tmeas2=125 C  EG_param=1  EG=1.11 eV  XTI_param=1  XTI=3  dBVdT=0 V/K  Tdevice=25 C  Rth=[ 0 10 ] K/W  thermal_mass_parameterization=1  thermal_mass=[ 0 1 ] J/K  thermal_time_constant=[ 0 10 ] s  thermal_mass_initial_temperatures=[ 25 25 ] C
  Gain : Gain  Gain=7.34/1000
  Simulink-PS Converter1 : nesl_utility/Simulink-PS Converter  PhysicalDomain=network_engine_domain  SubClassName=ps_input  LeftPortType=input  RightPortType=output  PseudoPeriodic=off  Frequencies=[]  NoiseDistribution=none  NoiseParameters=[]  Unit=1  AffineConversion=off  InputFiltering=off  SimscapeFilterOrder=1  InputFilterTimeConstant=0.001  UdotUserProvided=1
  + : PMIOPort  Port=1  Side=Right
  - : PMIOPort  Port=2  Side=Right
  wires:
  G/1 -> Gain/1
  Gain/1 -> Simulink-PS Converter1/1
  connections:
  Simulink-PS Converter1/RConn1 -- Controlled Current Source/RConn1
  Diode/RConn1 -- -/RConn1 -- Controlled Current Source/RConn2
  Diode/LConn1 -- Controlled Current Source/LConn1 -- +/RConn1

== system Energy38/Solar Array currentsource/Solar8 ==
  G : Inport
  Controlled Current Source : fl_lib/Electrical/Electrical Sources/Controlled Current Source
  Diode : elec_lib/Semiconductor Devices/Diode  ModelType=3  Vf=0.6 V  Ron=0.3 Ohm  Goff=1e-8 S  Rz=0.3 Ohm  Vz=50 V  C_PWL=5 pF  prmExp=2  I12=[ 0.0137 0.545 ] A  V12=[ 0.6 0.7 ] V  I1=0.0137 A  V1=0.6 V  RS=0.01 Ohm  IS=1.2614e-07 A  Tmeas=25 C  ec=117.5087  BV=Inf V  C_param=1  CJ0=5 pF  VJ=1 V  Mgrad=0.5  Vvec=[ 0.1 10 100 ] V  Cvec=[ 3.5 1 0.4 ] pF  FC=0.5  Q_param=1  Irrm=-7.15 A  iF=4 A  didt=-750 A/us  trr=115 ns  TT=50 ns  tau=100 ns  T_param=1  IS_T2=1.25e-7 A  I1_T2=0.245 A  V1_T2=0.5 V  Tmeas2=125 C  EG_param=1  EG=1.11 eV  XTI_param=1  XTI=3  dBVdT=0 V/K  Tdevice=25 C  Rth=[ 0 10 ] K/W  thermal_mass_parameterization=1  thermal_mass=[ 0 1 ] J/K  thermal_time_constant=[ 0 10 ] s  thermal_mass_initial_temperatures=[ 25 25 ] C
  Gain : Gain  Gain=7.34/1000
  Simulink-PS Converter1 : nesl_utility/Simulink-PS Converter  PhysicalDomain=network_engine_domain  SubClassName=ps_input  LeftPortType=input  RightPortType=output  PseudoPeriodic=off  Frequencies=[]  NoiseDistribution=none  NoiseParameters=[]  Unit=1  AffineConversion=off  InputFiltering=off  SimscapeFilterOrder=1  InputFilterTimeConstant=0.001  UdotUserProvided=1
  + : PMIOPort  Port=1  Side=Right
  - : PMIOPort  Port=2  Side=Right
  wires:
  G/1 -> Gain/1
  Gain/1 -> Simulink-PS Converter1/1
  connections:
  Simulink-PS Converter1/RConn1 -- Controlled Current Source/RConn1
  Diode/RConn1 -- -/RConn1 -- Controlled Current Source/RConn2
  Diode/LConn1 -- Controlled Current Source/LConn1 -- +/RConn1

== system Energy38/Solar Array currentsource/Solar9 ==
  G : Inport
  Controlled Current Source : fl_lib/Electrical/Electrical Sources/Controlled Current Source
  Diode : elec_lib/Semiconductor Devices/Diode  ModelType=3  Vf=0.6 V  Ron=0.3 Ohm  Goff=1e-8 S  Rz=0.3 Ohm  Vz=50 V  C_PWL=5 pF  prmExp=2  I12=[ 0.0137 0.545 ] A  V12=[ 0.6 0.7 ] V  I1=0.0137 A  V1=0.6 V  RS=0.01 Ohm  IS=1.2614e-07 A  Tmeas=25 C  ec=117.5087  BV=Inf V  C_param=1  CJ0=5 pF  VJ=1 V  Mgrad=0.5  Vvec=[ 0.1 10 100 ] V  Cvec=[ 3.5 1 0.4 ] pF  FC=0.5  Q_param=1  Irrm=-7.15 A  iF=4 A  didt=-750 A/us  trr=115 ns  TT=50 ns  tau=100 ns  T_param=1  IS_T2=1.25e-7 A  I1_T2=0.245 A  V1_T2=0.5 V  Tmeas2=125 C  EG_param=1  EG=1.11 eV  XTI_param=1  XTI=3  dBVdT=0 V/K  Tdevice=25 C  Rth=[ 0 10 ] K/W  thermal_mass_parameterization=1  thermal_mass=[ 0 1 ] J/K  thermal_time_constant=[ 0 10 ] s  thermal_mass_initial_temperatures=[ 25 25 ] C
  Gain : Gain  Gain=7.34/1000
  Simulink-PS Converter1 : nesl_utility/Simulink-PS Converter  PhysicalDomain=network_engine_domain  SubClassName=ps_input  LeftPortType=input  RightPortType=output  PseudoPeriodic=off  Frequencies=[]  NoiseDistribution=none  NoiseParameters=[]  Unit=1  AffineConversion=off  InputFiltering=off  SimscapeFilterOrder=1  InputFilterTimeConstant=0.001  UdotUserProvided=1
  + : PMIOPort  Port=1  Side=Right
  - : PMIOPort  Port=2  Side=Right
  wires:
  G/1 -> Gain/1
  Gain/1 -> Simulink-PS Converter1/1
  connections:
  Simulink-PS Converter1/RConn1 -- Controlled Current Source/RConn1
  Diode/RConn1 -- -/RConn1 -- Controlled Current Source/RConn2
  Diode/LConn1 -- Controlled Current Source/LConn1 -- +/RConn1
